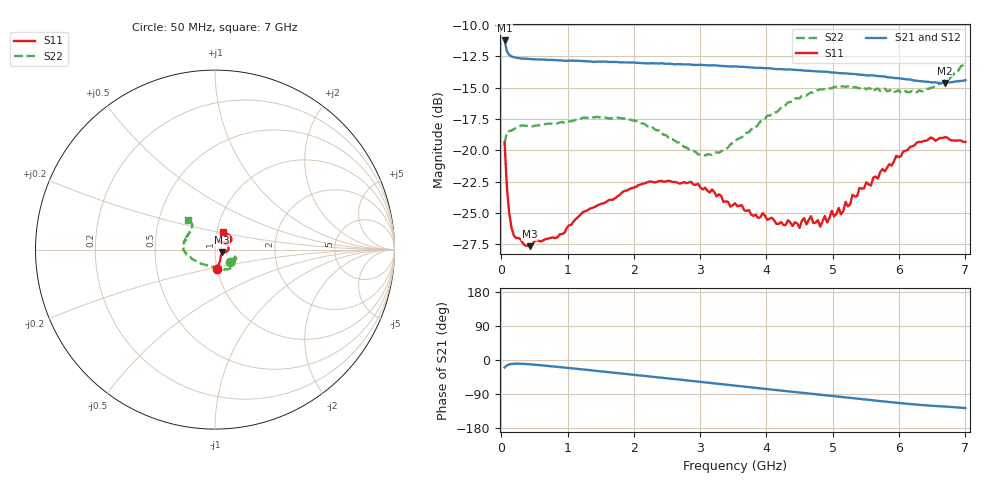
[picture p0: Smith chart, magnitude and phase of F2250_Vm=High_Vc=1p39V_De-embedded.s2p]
! Integrated Device Technology
! Corporate Headquarters
! 6024 Silver Creek Valley Road
! San Jose, CA 95138  USA
! Phone:  1-408-284-8200
! Toll Free:  1-800-223-1366
! Webpage:  http://www.idt.com/
! Timing and RF Division
! 515 Groton Road, Suite 102
! Westford, MA 01886-6024
! Device:  F2250
! Description: Voltage Variable RF Attenuator
! Frequency:  50.0 -  6000.00 MHz
! Package:  3x3 mm Thin QFN Plastic Package: 16 pin
! Ports:  2 RF, 3 DC
!  Pin  1  = GND
!  Pin  2  = NC
!  Pin  3  = RF1  = Port 1
!  Pin  4  = NC
!  Pin  5  = GND
!  Pin  6  = GND
!  Pin  7  = GND
!  Pin  8  = GND
!  Pin  9  = NC
!  Pin 10  = RF2  = Port 2
!  Pin 11  = NC
!  Pin 12  = GND
!  Pin 13  = GND
!  Pin 14  = VCNTRL
!  Pin 15  = VDD
!  Pin 16  = VMODE
! Vcntrl:  1.390 Volts
! Vmode:  +3.300 Volts
! Vdd:  +3.30  Volts
! Current:  1.330 mA
! Data:  The device was measured on a the F2250 evaluation board which has
!  individual transmission lines to the RF pins.  Data was collected
!  using a calibrated network analyzer.  The evaluation board was
!  de-embedded using a TRL calibration technique.
!  The reference plane is the edge of the package pin.
! Misc:  SN 10
!  Action Tracker AT0258
! Date Measured:  2014-11-26
! Date:  2015-10-15  MJV
! Note:
!  Integrated Device Technology supplies this data as a sample of measured
!  data at the package pin for this product.  Your particular data for this
!  product may vary.
!  Data was taken at 25 degrees C.
!  Integrated Device Technology reserves the right to change this data at anytime.
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# GHz S dB R 50
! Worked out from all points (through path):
!   201 points, 50 MHz to 7 GHz, reference 50 ohm
!   highest |S21| = -11.22 dB at 50 MHz (marker M1); lowest = -14.6 dB at 6.687 GHz (marker M2)
!   group delay of S21, straight-line fit = 50.2 ps
!   lowest |S11| = -27.6 dB at 432.2 MHz (marker M3), VSWR 1.09, Z = 54 - j1.73 ohm
!   |S11| at or under -10 dB: start of sweep to end of sweep
!   |S22| runs from -20.4 to -13.0 dB; largest |S21 - S12| = 0.0012
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0.05  -19.36 -85.0  -11.22 -19.6  -11.22 -19.5  -19.41 -40.4
0.08475  -22.98 -66.6  -12.09 -14.1  -12.08 -14.1  -18.55 -21.9
0.15425  -26.16 -49.0  -12.50 -10.5  -12.49 -10.4  -18.42 -14.8
0.43225  -27.64 -22.7  -12.70 -11.4  -12.71 -11.4  -18.05 -17.0
0.9535  -26.58 -20.1  -12.85 -19.9  -12.84 -20.0  -17.82 -33.8
1.2315  -24.92 -16.5  -12.88 -24.9  -12.87 -24.9  -17.39 -40.8
2.37825  -22.45 3.9  -13.06 -45.9  -13.07 -45.9  -18.38 -66.5
3.07325  -22.97 23.6  -13.19 -59.0  -13.19 -59.0  -20.41 -102.4
3.525  -24.22 39.5  -13.29 -67.6  -13.31 -67.6  -19.29 -133.2
4.1505  -25.87 59.2  -13.51 -79.3  -13.50 -79.4  -16.95 -161.9
4.498  -26.18 57.5  -13.59 -85.9  -13.61 -85.9  -15.84 -172.4
4.67175  -25.25 57.6  -13.66 -89.2  -13.68 -89.2  -15.37 -176.1
4.7065  -25.80 58.2  -13.68 -89.8  -13.68 -89.8  -15.39 -176.7
4.88025  -25.23 51.3  -13.72 -93.2  -13.72 -93.2  -15.10 179.4
4.915  -25.75 50.8  -13.72 -93.8  -13.74 -93.8  -15.04 178.6
5.08875  -24.58 45.0  -13.83 -97.0  -13.83 -97.0  -14.99 174.9
5.1235  -25.10 45.0  -13.84 -97.7  -13.81 -97.7  -14.92 173.9
5.193  -24.10 40.2  -13.85 -98.9  -13.84 -99.0  -14.94 172.6
5.85325  -21.09 27.8  -14.17 -110.9  -14.18 -111.0  -15.24 155.5
6.27025  -19.36 31.1  -14.44 -117.7  -14.43 -117.8  -15.35 142.4
6.68725  -18.95 44.9  -14.62 -122.8  -14.60 -123.0  -14.43 132.1
7  -19.32 67.0  -14.40 -127.0  -14.43 -127.0  -12.98 132.7
